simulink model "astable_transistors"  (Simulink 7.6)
settings: Solver=ode15s  StartTime=0.0  StopTime=0.03  RelTol=1e-3
InitFcn:
  | clear all, clc
libraries: fl_lib x11, nesl_utility x5, elec_lib x3, gaugeslibv2 x1

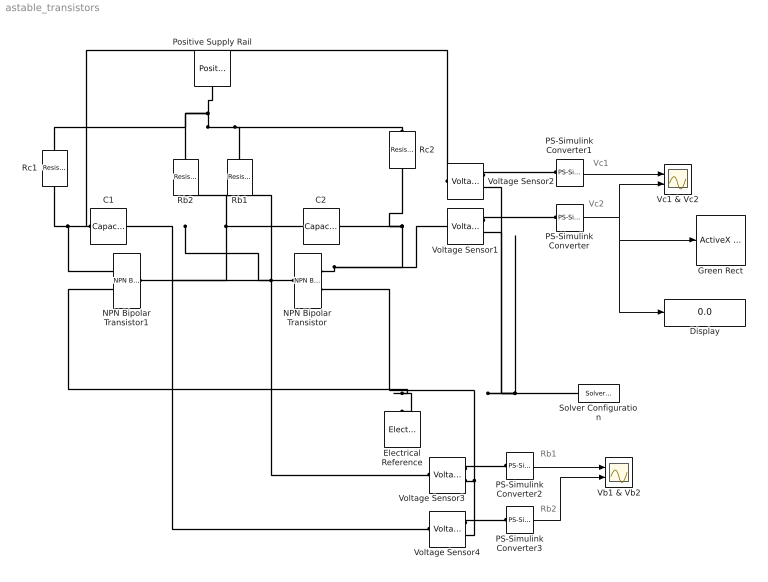
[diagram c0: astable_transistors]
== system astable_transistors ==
  note: Vc1
  note: Vc2
  note: Rb2
  note: Rb1
  C1 : fl_lib/Electrical/Electrical Elements/Capacitor  DialogController=NetworkEngine.DynNeDlgSource  SystemSampleTime=-1  c=0.01 uF  v0=0 V  r=1e-12 Ohm  g=0 1/Ohm  i_Log=off  v_Log=off  vc_Log=off  LocalVarNames=|i|v|vc  LocalVarDescs=|i|v|Internal variable for voltage across capacitor term  LocalVarLogging=[0 0 0]
  C2 : fl_lib/Electrical/Electrical Elements/Capacitor  DialogController=NetworkEngine.DynNeDlgSource  SystemSampleTime=-1  c=0.01 uF  v0=5 V  r=1e-12 Ohm  g=0 1/Ohm  i_Log=off  v_Log=off  vc_Log=off  LocalVarNames=|i|v|vc  LocalVarDescs=|i|v|Internal variable for voltage across capacitor term  LocalVarLogging=[0 0 0]
  Display : Display
  Electrical Reference : fl_lib/Electrical/Electrical Elements/Electrical Reference  DialogController=NetworkEngine.DynNeDlgSource  SystemSampleTime=-1  i_Log=off  LocalVarNames=|i  LocalVarDescs=|i  LocalVarLogging=0
  Green Rect : gaugeslibv2/ActiveX Control  progid=MWLED.ledctrl.1  connect=input  input=Value  init=hActx.configuration='LED\Individual\Green Rectangle';hActx.value=1;hActx.Mode=0;hActx.MouseControl=0;  inblock=on  border=on  updateParam=0
  NPN Bipolar Transistor : elec_lib/Semiconductor Devices/NPN Bipolar Transistor  DialogController=NetworkEngine.DynNeDlgSource  SystemSampleTime=-1  parameterization=1  BF=100  IS=1e-14 A  VAF=200 V  hfe=100  hoe=5e-5 1/Ohm  Ic_h=1 mA  V1=0.55 V  I1=0.5 mA  BR=1  Tmeas=25 C  RC=0.01 Ohm  RE=1e-4 Ohm  RB=1 Ohm  C_BC=5 pF  C_BE=5 pF  TF=0 us  TR=0 us  LocalVarLogging=[]
  NPN Bipolar Transistor1 : elec_lib/Semiconductor Devices/NPN Bipolar Transistor  DialogController=NetworkEngine.DynNeDlgSource  SystemSampleTime=-1  parameterization=1  BF=100  IS=1e-14 A  VAF=200 V  hfe=100  hoe=5e-5 1/Ohm  Ic_h=1 mA  V1=0.55 V  I1=0.5 mA  BR=1  Tmeas=25 C  RC=0.01 Ohm  RE=1e-4 Ohm  RB=1 Ohm  C_BC=5 pF  C_BE=5 pF  TF=0 us  TR=0 us  LocalVarLogging=[]
  PS-Simulink Converter{,1..3} (4 alike) : nesl_utility/PS-Simulink Converter  DialogController=NetworkEngine.DynNeUtilDlgSource  SystemSampleTime=-1  PhysicalDomain=network_engine_domain  LeftPortType=input  RightPortType=output  SubClassName=ps_output  Unit=1  AffineConversion=off
  Positive Supply Rail : elec_lib/Sources/Positive Supply Rail  DialogController=NetworkEngine.DynNeDlgSource  SystemSampleTime=-1  v0=5 V  current_Log=off  voltage_Log=off  power_Log=off  LocalVarNames=|current|voltage|power  LocalVarDescs=|Current (A)|Voltage (V)|Power (W)  LocalVarLogging=[0 0 0]
  Rb1 : fl_lib/Electrical/Electrical Elements/Resistor  DialogController=NetworkEngine.DynNeDlgSource  SystemSampleTime=-1  R=330 kOhm  i_Log=off  v_Log=off  LocalVarNames=|i|v  LocalVarDescs=|i|v  LocalVarLogging=[0 0]
  Rb2 : fl_lib/Electrical/Electrical Elements/Resistor  DialogController=NetworkEngine.DynNeDlgSource  SystemSampleTime=-1  R=330 kOhm  i_Log=off  v_Log=off  LocalVarNames=|i|v  LocalVarDescs=|i|v  LocalVarLogging=[0 0]
  Rc1 : fl_lib/Electrical/Electrical Elements/Resistor  DialogController=NetworkEngine.DynNeDlgSource  SystemSampleTime=-1  R=3 kOhm  i_Log=off  v_Log=off  LocalVarNames=|i|v  LocalVarDescs=|i|v  LocalVarLogging=[0 0]
  Rc2 : fl_lib/Electrical/Electrical Elements/Resistor  DialogController=NetworkEngine.DynNeDlgSource  SystemSampleTime=-1  R=3 kOhm  i_Log=off  v_Log=off  LocalVarNames=|i|v  LocalVarDescs=|i|v  LocalVarLogging=[0 0]
  Solver Configuration : nesl_utility/Solver Configuration  DialogController=NetworkEngine.DynNeUtilDlgSource  SystemSampleTime=-1  PhysicalDomain=network_engine_domain  LeftPortType=input  RightPortType=generic  SubClassName=solver  Accelerate=off  Profile=off  ResidualTolerance=1e-9  MaxNonlinIter=12  MaxModeIter=2  DoFixedCost=off  UseLocalSampling=off  DoDC=off  LinearAlgebra=Sparse  LocalSolverSampleTime=.001  LocalSolverChoice=NE_BACKWARD_EULER_ADVANCER  UseLocalSolver=off
  Vb1 & Vb2 : Scope  NumInputPorts=2
  Vc1 & Vc2 : Scope  NumInputPorts=2
  Voltage Sensor{1..4} (4 alike) : fl_lib/Electrical/Electrical Sensors/Voltage Sensor  DialogController=NetworkEngine.DynNeDlgSource  SystemSampleTime=-1  i1_Log=off  v1_Log=off  LocalVarNames=|i1|v1  LocalVarDescs=|i1|v1  LocalVarLogging=[]
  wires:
  PS-Simulink Converter/1 -> Display/1, Green Rect/1, Vc1 & Vc2/2
  PS-Simulink Converter1/1 -> Vc1 & Vc2/1
  PS-Simulink Converter2/1 -> Vb1 & Vb2/1
  PS-Simulink Converter3/1 -> Vb1 & Vb2/2
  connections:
  NPN Bipolar Transistor1/LConn1 -- Rb1/LConn1 -- C2/LConn1 -- Voltage Sensor4/LConn1
  C1/LConn1 -- Rb2/LConn1 -- NPN Bipolar Transistor/LConn1 -- Voltage Sensor3/LConn1
  NPN Bipolar Transistor/RConn1 -- Voltage Sensor1/LConn1 -- Rc2/LConn1 -- C2/RConn1
  C1/RConn1 -- Rc1/LConn1 -- NPN Bipolar Transistor1/RConn1 -- Voltage Sensor2/LConn1
  Voltage Sensor1/RConn1 -- PS-Simulink Converter/LConn1
  Rc2/RConn1 -- Positive Supply Rail/RConn1 -- Rc1/RConn1 -- Rb2/RConn1 -- Rb1/RConn1
  Voltage Sensor3/RConn2 -- Voltage Sensor1/RConn2 -- Voltage Sensor2/RConn2 -- Solver Configuration/RConn1 -- NPN Bipolar Transistor/RConn2 -- NPN Bipolar Transistor1/RConn2 -- Electrical Reference/LConn1 -- Voltage Sensor4/RConn2
  Voltage Sensor2/RConn1 -- PS-Simulink Converter1/LConn1
  Voltage Sensor3/RConn1 -- PS-Simulink Converter2/LConn1
  Voltage Sensor4/RConn1 -- PS-Simulink Converter3/LConn1
